TYPE "KOM Ext->Sw"
TITLE =Kommunikationssignale von Extern
AUTHOR : dfb
FAMILY : KOM
NAME : 'AP&TSw'
VERSION : 0.1


  STRUCT
IN: STRUCT //Eingangssignale
LifeBit : Bool ;  //Life bit communication
EmStopLineOK : Bool ;  //Emergency stop line OK
GuardsZon1OK : Bool ;  //Guards press cell OK
GuardsZon2OK : Bool ;  //Guards loading furnace OK
Spare_0_4 : Bool ;  //Reserve
Spare_0_5 : Bool ;  //Reserve
Spare_0_6 : Bool ;  //Reserve
Spare_0_7 : Bool ;  //Reserve
CycleStopReqZ1 : Bool ;  //Request cycle stop (open guards) press cell
CycleStopReqZ2 : Bool ;  //Request cycle stop (open guards) zone loading furance
ReqOpModeAuto : Bool ;  //Request operation mode Auto
AutoStartOn : Bool ;  //Automatic start
ReqChangeRecipe : Bool ;  //Request change recipe
Spare_1_5 : Bool ;  //Reserve
Spare_1_6 : Bool ;  //Reserve
Rob2_left_part : Bool ;  //Robot has leaved parts
SF_RequestPart : Bool ;  //Request new part/parts from furnace
SF_ReadyForPart2 : Bool ;  //SF ready for part 2
SF_ReadyForPart3 : Bool ;  //SF ready for part 3
SF_ReadyForPart4 : Bool ;  //SF ready for part 4
SF_PartPicked : Bool ;  //SF has picked parts
Spare_2_5 : Bool ;  //Reserve
Spare_2_6 : Bool ;  //Reserve
Spare_2_7 : Bool ;  //Reserve
Spare_3_0 : Bool ;  //Reserve
Spare_3_1 : Bool ;  //Reserve
Spare_3_2 : Bool ;  //Reserve
Spare_3_3 : Bool ;  //Reserve
Spare_3_4 : Bool ;  //Reserve
Spare_3_5 : Bool ;  //Reserve
Spare_3_6 : Bool ;  //Reserve
Spare_3_7 : Bool ;  //Reserve
Spare_4_0 : Bool ;  //Reserve
Spare_4_1 : Bool ;  //Reserve
Spare_4_2 : Bool ;  //Reserve
Spare_4_3 : Bool ;  //Reserve
Spare_4_4 : Bool ;  //Reserve
Spare_4_5 : Bool ;  //Reserve
Spare_4_6 : Bool ;  //Reserve
Spare_4_7 : Bool ;  //Reserve
Spare_5_0 : Bool ;  //Reserve
Spare_5_1 : Bool ;  //Reserve
Spare_5_2 : Bool ;  //Reserve
Spare_5_3 : Bool ;  //Reserve
Spare_5_4 : Bool ;  //Reserve
Spare_5_5 : Bool ;  //Reserve
Spare_5_6 : Bool ;  //Reserve
Spare_5_7 : Bool ;  //Reserve
RecipeNo : INT ;  //RecipeNumber
Spare_8_0 : INT ;  //Reserve
END_STRUCT ;
END_STRUCT ;
END_TYPE
